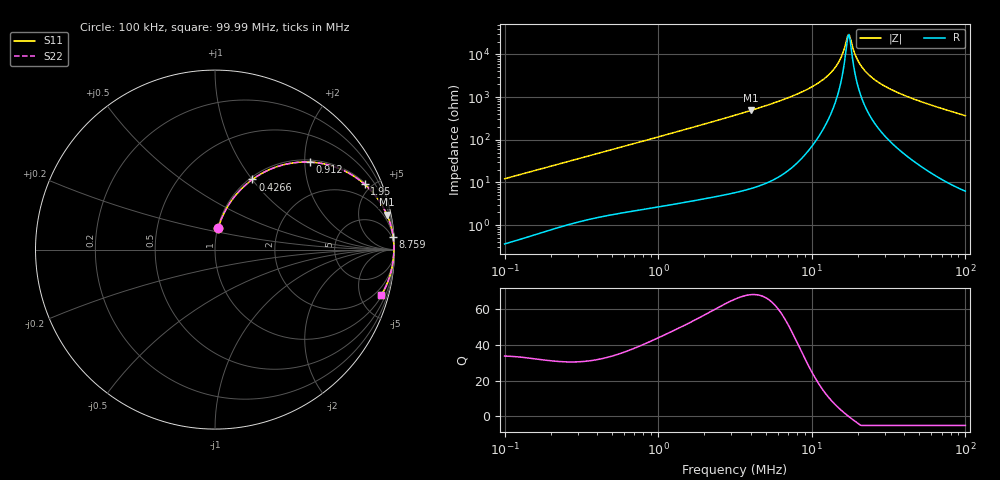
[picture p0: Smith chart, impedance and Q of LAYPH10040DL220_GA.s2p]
! LAYPH10040DL220_GA  S-PARAMETER MODEL  ( General Type )
! Model Generated by TAIYO YUDEN Corporation (http://www.ty-top.com)
! Version 1.0
! TAIYO YUDEN Control No. 180920NI43SB-FBB
! Copyright(c) 2018 TAIYO YUDEN CO.,LTD. All Rights Reserved.
! Product Description (link to TY-COMPAS)
! https://ds.yuden.co.jp/TYCOMPAS/or/detail?pn=LAYPH10040DL220MGA&u=M
! Products Name : Inductors
! Characteristics :
!  Inductance : 22 uH , SRF(min) : -Hz , DC Resistance(max) : 0.074 Ohm
!  Rated Current : Saturation :2.5 A , Temp Rise : 1.5 A (25 degC)
!  Case Size : 10.1 x 10.0 / 0.398 x 0.394 [mm/inch] , Thickness : 4 / 0.157 [mm/inch]
!  (Conditions: Temperature = 25 degC , DC Bias Current/Voltage = 0A / 0V)
! External Node Assignments :
!  1  o---GGG---o  2
! GND o---------o GND
! Frequency Range : 0.1MHz  -  99.992428MHz  [ 402 STEP ]
# MHz S RI R 50
! Freq[MHz].  S11 Real  S11 Imag  S21 Real  S21 Imag  S12 Real  S12 Imag  S22 Real  S22 Imag
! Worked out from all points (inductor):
!   401 points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, 100 kHz to 99.99 MHz, reference 50 ohm
!   read as one part in series: L = 19.3 uH near 103.5 kHz
!   highest Q = 68 at 4.027 MHz (marker M1), where L = 19.3 uH
!   self-resonance near 17.18 MHz
!   S11 on the Smith chart (normalised r, x): 100 kHz: 1.01, +0.24; 426.6 kHz: 1.03, +1.00; 912 kHz: 1.05, +2.12; 1.95 MHz: 1.08, +4.54; 8.759 MHz: 2, +27; 99.99 MHz: 1.12, -7.33
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0.1  0.018 0.1188  0.982 -0.1188  0.982 -0.1188  0.018 0.1188
0.318049  0.1325 0.3231  0.8675 -0.3231  0.8675 -0.3231  0.1325 0.3231
0.426573  0.2087 0.3912  0.7913 -0.3912  0.7913 -0.3912  0.2087 0.3912
0.911989  0.5289 0.4875  0.4711 -0.4875  0.4711 -0.4875  0.5289 0.4875
1.011554  0.5786 0.4826  0.4214 -0.4826  0.4214 -0.4826  0.5786 0.4826
1.949781  0.8333 0.3639  0.1667 -0.3639  0.1667 -0.3639  0.8333 0.3639
3.162158  0.9304 0.247  0.0696 -0.247  0.0696 -0.247  0.9304 0.247
4.027007  0.957 0.1955  0.043 -0.1955  0.043 -0.1955  0.957 0.1955
8.759488  0.9925 0.0729  0.00749 -0.0729  0.00749 -0.0729  0.9925 0.0729
10.05722  0.9945 0.0565  0.00554 -0.0565  0.00554 -0.0565  0.9945 0.0565
12.16122  0.996 0.0358  0.00398 -0.0358  0.00398 -0.0358  0.996 0.0358
13.96293  0.9966 0.0216  0.00344 -0.0216  0.00344 -0.0216  0.9966 0.0216
15.22215  0.9967 0.013  0.00331 -0.013  0.00331 -0.013  0.9967 0.013
16.88401  0.9967 0.00287  0.00331 -0.00287  0.00331 -0.00287  0.9967 0.00287
17.47734  0.9966 -0.00049  0.00336 0.00049  0.00336 0.00049  0.9966 -0.00049
17.78178  0.9966 -0.00217  0.00338 0.00217  0.00338 0.00217  0.9966 -0.00217
19.72309  0.9963 -0.0122  0.00365 0.0122  0.00365 0.0122  0.9963 -0.0122
21.50178  0.996 -0.0207  0.00401 0.0207  0.00401 0.0207  0.996 -0.0207
25.11734  0.995 -0.0364  0.00502 0.0364  0.00502 0.0364  0.995 -0.0364
31.98693  0.9923 -0.0624  0.0077 0.0624  0.0077 0.0624  0.9923 -0.0624
50.98828  0.9806 -0.1235  0.0194 0.1235  0.0194 0.1235  0.9806 -0.1235
99.99243  0.927 -0.2518  0.073 0.2518  0.073 0.2518  0.927 -0.2518
